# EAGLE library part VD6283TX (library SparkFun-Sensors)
Hybrid filter multispectral sensor with light flicker engine VD6283TX light measurement is fast and accurate thanks to an individual ADC and a readout for each color channel. It employs hybrid color filters with precise responses allowing accurate computation of the correlated color temperature (CCT) and Lux information. The VD6283TX can be used for display brightness management or scene light correction and can extract light flickering frequencies to avoid “banding effects” on videos, or check that they are safe for human eye. Additionally, the VD6283TX is the only sensor able to extract different light flicker waveforms from 100 Hz and 2 kHz, including LED square signals, that can run flicker operations simultaneously with ALS operations.
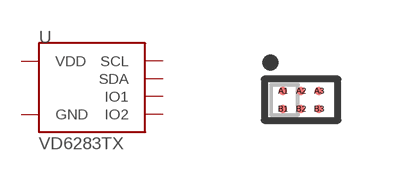
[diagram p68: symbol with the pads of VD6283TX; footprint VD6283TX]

Designator prefix U

## VD6283TX (PROD_ID: IC-16459)  [VD6283TX]
A1  VDD  pwr
A2  SDA
A3  GND  pwr
B1  IO2
B2  IO1
B3  SCL

## Footprint VD6283TX (pad centres in mm)
smd 0.21 x 0.21: A1 -0.45,0.225; A2 0,0.225; A3 0.45,0.225; B1 -0.45,-0.225; B2 0,-0.225; B3 0.45,-0.225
